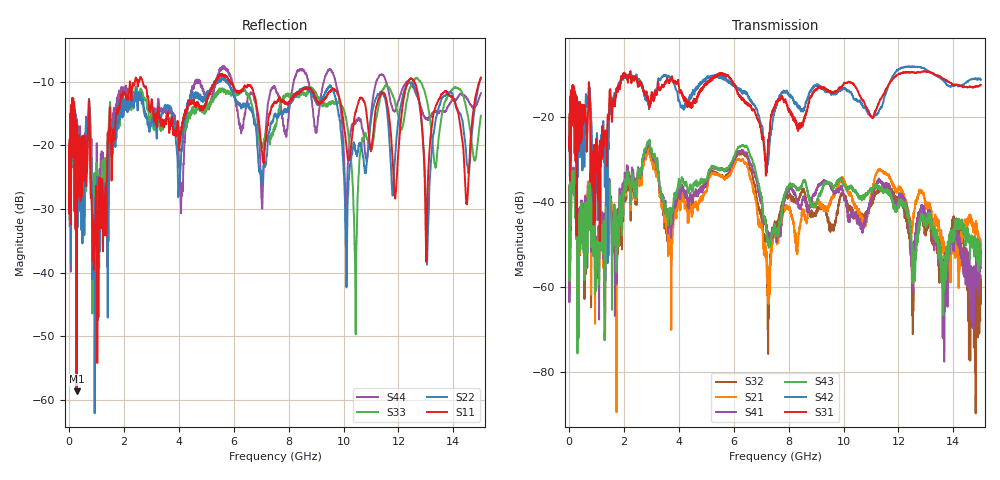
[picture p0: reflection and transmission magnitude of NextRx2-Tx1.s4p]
! FILE: N:\QM 2007\Prüfprotokolle\Highspeed\Konfektionierte Ltg\L45593-D106\D30\8216\0002\Next  Platine 2\NextRx2-Tx1.s4p
# MHz S DB R 50.00
! FREQ  S11  S12  S13  S14
!  S21  S22  S23  S24
!  S31  S32  S33  S34
!  S41  S42  S43  S44
!  DB  ANG  DB  ANG  DB  ANG  DB  ANG
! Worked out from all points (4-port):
!   2999 points, 10 MHz to 15 GHz, reference 50 ohm
!   strongest paths, dB at 10 MHz, 3.755 GHz, 7.505 GHz, 11.26 GHz, 15 GHz:
!     S31: -24.9, -10.5, -17.4, -17.1, -12.5
!     S42: -25.3, -11.4, -18.5, -19.2, -11.3
!     S43: -46.1, -42.0, -46.2, -36.3, -52.8
!     S41: -55.9, -44.3, -45.7, -35.5, -55.7
!     S21: -55.9, -49.0, -46.9, -32.8, -50.3
!     S32: -48.1, -45.9, -46.1, -37.5, -58.5
!   lowest |S11| = -58.6 dB at 280 MHz (marker M1), VSWR 1.00, Z = 49.9 + j0.1 ohm
!   |S11| at or under -10 dB: 2.69 GHz to 5.299 GHz (2.609 GHz wide, 65.3 % of centre); 5.886 GHz to 12.34 GHz (6.459 GHz wide, 70.9 % of centre); 12.58 GHz to 14.94 GHz (2.367 GHz wide, 17.2 % of centre)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
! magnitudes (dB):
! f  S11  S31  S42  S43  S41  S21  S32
! 10 MHz  -20.2  -24.9  -25.3  -46.1  -55.9  -55.9  -48.1
! 280 MHz  -58.6  -48.0  -30.8  -47.9  -46.6  -44.9  -46.9
! 6.32 GHz  -11.2  -16.0  -14.5  -26.8  -27.9  -30.1  -28.6
! 7.26 GHz  -16.0  -25.4  -30.5  -50.3  -48.6  -60.6  -62.9
! 10.43 GHz  -14.8  -13.0  -16.0  -37.3  -42.6  -41.0  -42.9
! 11.6 GHz  -13.7  -13.1  -13.6  -37.5  -35.6  -33.6  -36.4
! 15 GHz  -9.3  -12.5  -11.3  -52.8  -55.7  -50.3  -58.5
